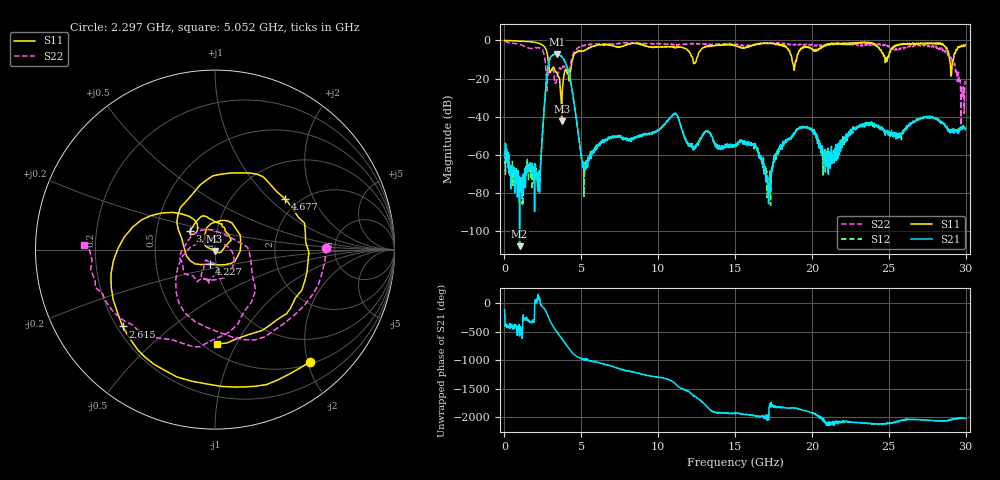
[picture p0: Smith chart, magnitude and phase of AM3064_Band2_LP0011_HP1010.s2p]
# Hz S DB R 50.0
!freq dBS11 angS11 dBS21 angS21 dBS12 angS12 dBS22 angS22
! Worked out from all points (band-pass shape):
!   1600 points, 10 MHz to 29.98 GHz, reference 50 ohm
!   highest |S21| = -7.07 dB at 3.403 GHz (marker M1); lowest = -107.8 dB at 984.7 MHz (marker M2)
!   |S21| within 3 dB of the highest: 2.929 GHz to 3.868 GHz (939.1 MHz wide, 27.6 % of centre)
!   lowest |S11| = -42.5 dB at 3.721 GHz (marker M3), VSWR 1.02, Z = 49.8 - j0.709 ohm
!   |S11| at or under -10 dB: 2.839 GHz to 4.435 GHz (1.595 GHz wide, 43.9 % of centre); 18.7 GHz to 19 GHz (298 MHz wide, 1.58 % of centre); 28.94 GHz to 29.2 GHz (255.7 MHz wide, 0.88 % of centre)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
!   |S22| runs from -44.5 to -0.2 dB; largest |S21 - S12| = 0.014
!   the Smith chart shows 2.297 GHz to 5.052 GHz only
!   S11 on the Smith chart (normalised r, x): 2.297 GHz: 0.54, -2.05; 2.615 GHz: 0.22, -0.35; 3.065 GHz: 0.74, +0.16; 4.227 GHz: 0.93, -0.15; 4.677 GHz: 1.71, +1.25; 5.052 GHz: 0.58, -0.84
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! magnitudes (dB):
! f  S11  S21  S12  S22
! 10 MHz  0.0  -58.3  -61.1  -0.2
! 984.7 MHz  -0.4  -107.8  -75.4  -2.1
! 2.297 GHz  -1.7  -78.6  -73.8  -4.2
! 2.615 GHz  -3.5  -32.2  -32.1  -8.8
! 3.065 GHz  -15.2  -8.1  -8.1  -15.4
! 3.403 GHz  -16.9  -7.1  -7.3  -20.3
! 3.721 GHz  -42.5  -8.5  -8.6  -13.8
! 4.227 GHz  -21.3  -18.6  -18.4  -15.7
! 4.677 GHz  -6.3  -41.3  -41.2  -4.8
! 5.015 GHz  -5.8  -60.4  -61.8  -3.3
! 5.052 GHz  -5.6  -63.0  -63.2  -2.7
! 10 GHz  -3.5  -46.7  -46.8  -1.8
! 15 GHz  -2.6  -54.6  -54.3  -1.9
! 16.32 GHz  -2.2  -54.5  -54.5  -2.0
! 17.18 GHz  -1.8  -85.5  -79.7  -1.5
! 18.04 GHz  -2.5  -57.1  -54.9  -1.9
! 19.99 GHz  -4.2  -47.2  -47.3  -2.1
! 21.21 GHz  -2.2  -61.0  -58.8  -2.1
! 23.12 GHz  -1.3  -45.0  -44.1  -2.8
! 25 GHz  -8.2  -47.6  -48.2  -2.8
! 28.56 GHz  -2.5  -43.5  -43.4  -4.7
! 29.98 GHz  -2.3  -46.2  -47.6  -21.6
